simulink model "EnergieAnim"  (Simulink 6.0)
settings: Solver=ode45  StartTime=0.0  StopTime=SimTime  FixedStep=1E-2  RelTol=1e-5
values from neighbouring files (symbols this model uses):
  b = S/Sm    (= 0.1)    [Constantes.m]    (also in ConstantesBck.m)
  beta = 1    [ResCourV1.m]    (also in ResCrV1.m; ResEnerV1.m; Constantes.m = 0.95; ConstantesBck.m = 0.95)
  C = 1    [Constantes.m]    (also in ConstantesBck.m)
  Cdl = 731.3E-9    (= 7.313e-07)    [ResCourV1.m]    (also in ResCrV1.m; ResEnerV1.m; Constantes.m = 6.03e-07; ConstantesBck.m = 6.03e-07)
  Cmem = 1E-6*Sm*(1-b)    (= 2.826e-08)    [Constantes.m]    (also in ConstantesBck.m = 3.14e-11; ImpedanceZtissus.m = 4e-08; Ztissus.m = 4e-08; CalculCharge.m = 1)
  Fact = 10^2    (= 100)    [Constantes.m]    (also in ConstantesBck.m)
  gk = 36    [Constantes.m]    (also in ConstantesBck.m; sim_hh.m)
  gl = 0.3    [Constantes.m]    (also in ConstantesBck.m; sim_hh.m)
  gna = 120    [Constantes.m]    (also in ConstantesBck.m; sim_hh.m)
  h0 = cdep(4)    [temps.m]    (also in Constantes.m = 0.5961; ConstantesBck.m = 0.5961)
  I0Stim = AddI    (= 0)    [WaveComp.m]    (also in WaveCompIET.m; WaveCompIETAnim.m; WaveCompIETIf.m; WaveCompIETSeul.m = Hm(i)*1E-6)
  m0 = cdep(5)    [temps.m]    (also in Constantes.m = 0.0529; ConstantesBck.m = 0.0529)
  mK = 0    [Constantes.m]    (also in ConstantesBck.m)
  mL = 0    [Constantes.m]    (also in ConstantesBck.m)
  mNa = 0    [Constantes.m]    (also in ConstantesBck.m)
  n0 = 0.3177    [Constantes.m]    (also in ConstantesBck.m)
  Rcan = 6.398E3*Sm*(1-b)    (= 180.80748)    [Constantes.m]    (also in ConstantesBck.m = 0.03454; ImpedanceZtissus.m = 44; Ztissus.m = 44)
  Rct = 605.2E3    (= 605200)    [ResCourV1.m]    (also in ResCrV1.m; ResEnerV1.m; Constantes.m = 185600; ConstantesBck.m = 185600)
  sigma = 68000    [ResCourV1.m]    (also in ResCrV1.m; ResEnerV1.m; Constantes.m = 66466; ConstantesBck.m = 66466)
  Sm = 3.14e-2    (= 0.0314)    [Constantes.m]    (also in ConstantesBck.m = 0.000314)
  T0Stim = i    [WaveComp.m]    (also in WaveCompIET.m; WaveCompIETAnim.m = 5; WaveCompIETIf.m; WaveCompIETSeul.m = T0Hm(i)*1E-3)
  TypeStim = 5    [WaveComp.m]    (also in WaveCompIET.m; WaveCompIETAnim.m; WaveCompIETIf.m; WaveCompIETSeul.m)
  Vk = -82    [Constantes.m]    (also in ConstantesBck.m)
  Vl = -59    [Constantes.m]    (also in ConstantesBck.m)
  Vna = 45    [Constantes.m]    (also in ConstantesBck.m)
  Vr = -70    [Constantes.m]    (also in ConstantesBck.m)
libraries: simulink x1

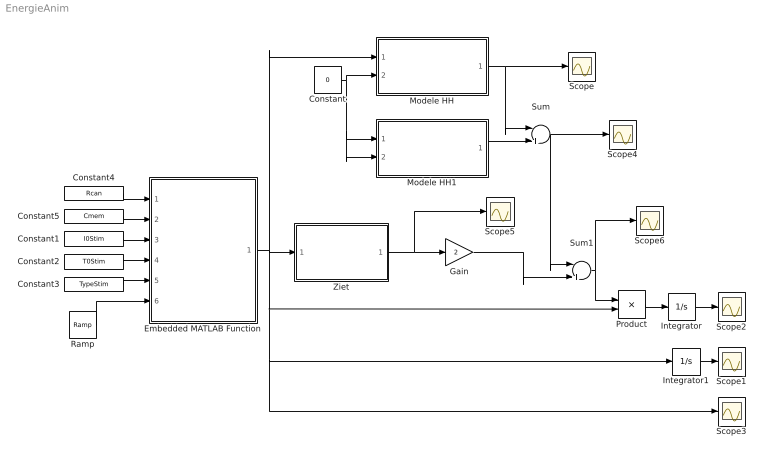
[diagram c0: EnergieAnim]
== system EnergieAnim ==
  Constant : Constant  Value=0
  Constant1 : Constant  Value=I0Stim
  Constant2 : Constant  Value=T0Stim
  Constant3 : Constant  Value=TypeStim
  Constant4 : Constant  Value=Rcan
  Constant5 : Constant  Value=Cmem
  Embedded MATLAB Function : Stateflow chart
  Gain : Gain  Gain=2
  Integrator : Integrator
  Integrator1 : Integrator
  Modele HH : Subsystem
  Modele HH1 : Subsystem
  Product : Product
  Ramp : simulink/Sources/Ramp  slope=1  start=0  X0=0
  Scope{,1..6} (7 alike) : Scope
  Sum : Sum  Inputs=|+-
  Sum1 : Sum  Inputs=|++
  Ziet : Subsystem
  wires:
  Product/1 -> Integrator/1
  Constant1/1 -> Embedded MATLAB Function/3(I0Stim)
  Constant2/1 -> Embedded MATLAB Function/4(T0Stim)
  Constant3/1 -> Embedded MATLAB Function/5(TypeStim)
  Ramp/1 -> Embedded MATLAB Function/6(temps)
  Embedded MATLAB Function/1(Istim) -> Product/2, Scope3/1, Integrator1/1, Modele HH/1(HHin), Ziet/1(InZiet)
  Constant4/1 -> Embedded MATLAB Function/1(Rcan)
  Constant5/1 -> Embedded MATLAB Function/2(Cmem)
  Modele HH/1(HHout) -> Scope/1, Sum/1
  Constant/1 -> Modele HH/2(VRefIn), Modele HH1/1(HHin), Modele HH1/2(VRefIn)
  Integrator/1 -> Scope2/1
  Modele HH1/1(HHout) -> Sum/2
  Sum/1 -> Sum1/1, Scope4/1
  Sum1/1 -> Product/1, Scope6/1
  Ziet/1(OutZiet) -> Gain/1, Scope5/1
  Gain/1 -> Sum1/2
  Integrator1/1 -> Scope1/1

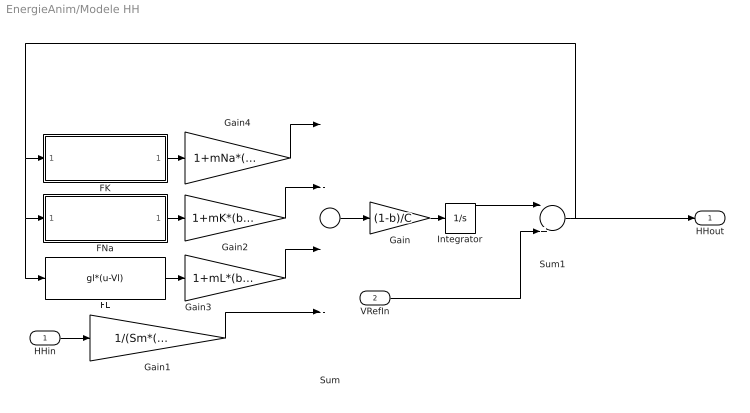
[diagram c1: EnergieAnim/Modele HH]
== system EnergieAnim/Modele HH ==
  HHin : Inport  Port=1  LatchInput=off
  VRefIn : Inport  Port=2  LatchInput=off
  FK : Subsystem
  FL : Fcn  Expr=gl*(u-Vl)
  FNa : Subsystem
  Gain : Gain  Gain=(1-b)/C
  Gain1 : Gain  Gain=1/(Sm*(1-b)*Fact)
  Gain2 : Gain  Gain=1+mK*(b/(1-b))
  Gain3 : Gain  Gain=1+mL*(b/(1-b))
  Gain4 : Gain  Gain=1+mNa*(b/(1-b))
  Integrator : Integrator  InitialCondition=Vr
  Sum : Sum  Inputs=|---+
  Sum1 : Sum  Inputs=|++
  HHout : Outport
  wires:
  Sum/1 -> Gain/1
  Gain/1 -> Integrator/1
  FK/1(FKout) -> Gain4/1
  FNa/1(FNaOut) -> Gain2/1
  FL/1 -> Gain3/1
  HHin/1 -> Gain1/1
  Integrator/1 -> Sum1/1
  Sum1/1 -> FNa/1(FNaIn), FL/1, FK/1(FKIn), HHout/1
  Gain1/1 -> Sum/4
  Gain4/1 -> Sum/1
  Gain2/1 -> Sum/2
  Gain3/1 -> Sum/3
  VRefIn/1 -> Sum1/2

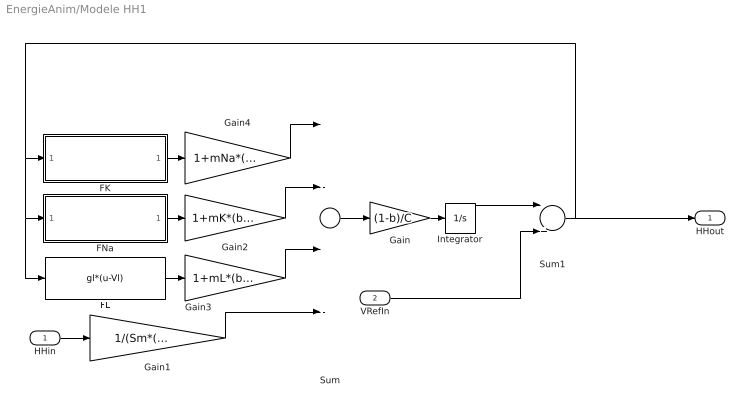
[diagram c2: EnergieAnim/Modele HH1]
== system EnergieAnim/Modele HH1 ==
  HHin : Inport  Port=1  LatchInput=off
  VRefIn : Inport  Port=2  LatchInput=off
  FK : Subsystem
  FL : Fcn  Expr=gl*(u-Vl)
  FNa : Subsystem
  Gain : Gain  Gain=(1-b)/C
  Gain1 : Gain  Gain=1/(Sm*(1-b)*Fact)
  Gain2 : Gain  Gain=1+mK*(b/(1-b))
  Gain3 : Gain  Gain=1+mL*(b/(1-b))
  Gain4 : Gain  Gain=1+mNa*(b/(1-b))
  Integrator : Integrator  InitialCondition=Vr
  Sum : Sum  Inputs=|---+
  Sum1 : Sum  Inputs=|++
  HHout : Outport
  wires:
  Sum/1 -> Gain/1
  Gain/1 -> Integrator/1
  FK/1(FKout) -> Gain4/1
  FNa/1(FNaOut) -> Gain2/1
  FL/1 -> Gain3/1
  HHin/1 -> Gain1/1
  Integrator/1 -> Sum1/1
  Sum1/1 -> FNa/1(FNaIn), FL/1, FK/1(FKIn), HHout/1
  Gain1/1 -> Sum/4
  Gain4/1 -> Sum/1
  Gain2/1 -> Sum/2
  Gain3/1 -> Sum/3
  VRefIn/1 -> Sum1/2

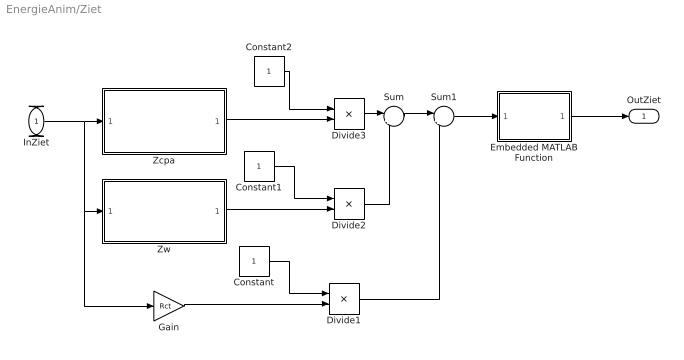
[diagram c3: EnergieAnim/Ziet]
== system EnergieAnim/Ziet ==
  InZiet : Inport  Port=1  LatchInput=off
  Constant : Constant
  Constant1 : Constant
  Constant2 : Constant
  Divide1 : Product  Inputs=*/  OutScaling=2^-10
  Divide2 : Product  Inputs=*/  OutScaling=2^-10
  Divide3 : Product  Inputs=*/  OutScaling=2^-10
  Embedded MATLAB Function : Stateflow chart
  Gain : Gain  Gain=Rct
  Sum : Sum  Inputs=|++
  Sum1 : Sum  Inputs=|++
  Zcpa : Subsystem
  Zw : Subsystem
  OutZiet : Outport
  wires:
  Constant/1 -> Divide1/1
  Constant1/1 -> Divide2/1
  Constant2/1 -> Divide3/1
  Zcpa/1(OutZcpa) -> Divide3/2
  Zw/1(OutZw) -> Divide2/2
  Divide3/1 -> Sum/1
  Divide2/1 -> Sum/2
  Sum/1 -> Sum1/1
  Divide1/1 -> Sum1/2
  Sum1/1 -> Embedded MATLAB Function/1(u)
  Gain/1 -> Divide1/2
  InZiet/1 -> Zcpa/1(InZcpa), Zw/1(InZw), Gain/1
  Embedded MATLAB Function/1(y) -> OutZiet/1

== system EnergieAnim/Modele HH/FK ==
  note: gkm
  note: (Vm-Vk0)
  FKIn : Inport  Port=1  LatchInput=off
  (Vm-Vk0) : Fcn  Expr=(u-Vk)
  Product : Product
  n(Vm) : Subsystem
  n^4 : Fcn  Expr=gk*(u^4)
  FKout : Outport  InitialOutput=0
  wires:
  n(Vm)/1(n) -> n^4/1
  (Vm-Vk0)/1 -> Product/2
  Product/1 -> FKout/1
  n^4/1 -> Product/1
  FKIn/1 -> n(Vm)/1(Vm), (Vm-Vk0)/1

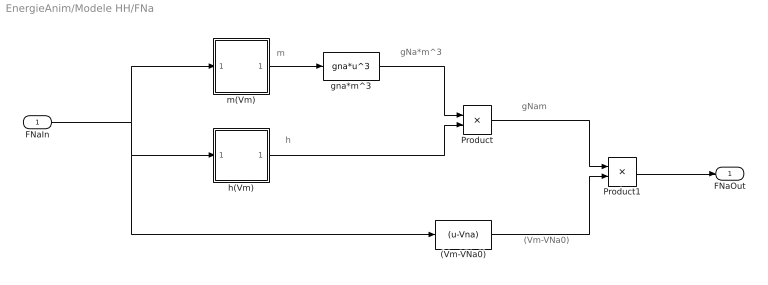
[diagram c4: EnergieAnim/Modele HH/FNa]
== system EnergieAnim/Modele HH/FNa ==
  note: gNa*m^3
  note: m
  note: h
  note: gNam
  note: (Vm-VNa0)
  FNaIn : Inport  Port=1  LatchInput=off
  (Vm-VNa0) : Fcn  Expr=(u-Vna)
  Product : Product
  Product1 : Product
  gna*m^3 : Fcn  Expr=gna*u^3
  h(Vm) : Subsystem
  m(Vm) : Subsystem
  FNaOut : Outport  InitialOutput=0
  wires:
  (Vm-VNa0)/1 -> Product1/2
  gna*m^3/1 -> Product/1
  Product1/1 -> FNaOut/1
  FNaIn/1 -> m(Vm)/1(Vm), h(Vm)/1(Vm), (Vm-VNa0)/1
  m(Vm)/1(n) -> gna*m^3/1
  h(Vm)/1(h) -> Product/2
  Product/1 -> Product1/1

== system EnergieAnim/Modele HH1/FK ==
  note: gkm
  note: (Vm-Vk0)
  FKIn : Inport  Port=1  LatchInput=off
  (Vm-Vk0) : Fcn  Expr=(u-Vk)
  Product : Product
  n(Vm) : Subsystem
  n^4 : Fcn  Expr=gk*(u^4)
  FKout : Outport  InitialOutput=0
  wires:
  n(Vm)/1(n) -> n^4/1
  (Vm-Vk0)/1 -> Product/2
  Product/1 -> FKout/1
  n^4/1 -> Product/1
  FKIn/1 -> n(Vm)/1(Vm), (Vm-Vk0)/1

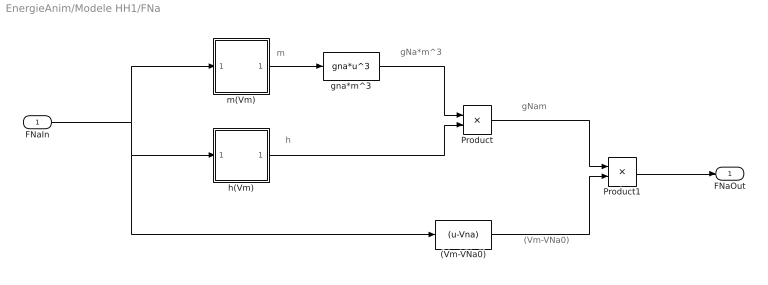
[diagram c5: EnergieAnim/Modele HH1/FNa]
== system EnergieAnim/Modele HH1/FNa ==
  note: gNa*m^3
  note: m
  note: h
  note: gNam
  note: (Vm-VNa0)
  FNaIn : Inport  Port=1  LatchInput=off
  (Vm-VNa0) : Fcn  Expr=(u-Vna)
  Product : Product
  Product1 : Product
  gna*m^3 : Fcn  Expr=gna*u^3
  h(Vm) : Subsystem
  m(Vm) : Subsystem
  FNaOut : Outport  InitialOutput=0
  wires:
  (Vm-VNa0)/1 -> Product1/2
  gna*m^3/1 -> Product/1
  Product1/1 -> FNaOut/1
  FNaIn/1 -> m(Vm)/1(Vm), h(Vm)/1(Vm), (Vm-VNa0)/1
  m(Vm)/1(n) -> gna*m^3/1
  h(Vm)/1(h) -> Product/2
  Product/1 -> Product1/1

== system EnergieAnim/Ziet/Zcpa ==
  InZcpa : Inport  Port=1  LatchInput=off
  Fcn : Fcn  Expr=u(1)^beta
  Transfer Fcn : TransferFcn  Denominator=[Cdl 0]
  OutZcpa : Outport
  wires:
  Transfer Fcn/1 -> Fcn/1
  InZcpa/1 -> Transfer Fcn/1
  Fcn/1 -> OutZcpa/1

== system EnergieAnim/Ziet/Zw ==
  InZw : Inport  Port=1  LatchInput=off
  Gain : Gain  Gain=sigma
  Math Function : Math  Operator=sqrt
  Transfer Fcn : TransferFcn  Numerator=[2]  Denominator=[1 0]
  OutZw : Outport
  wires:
  Transfer Fcn/1 -> Math Function/1
  Math Function/1 -> Gain/1
  Gain/1 -> OutZw/1
  InZw/1 -> Transfer Fcn/1

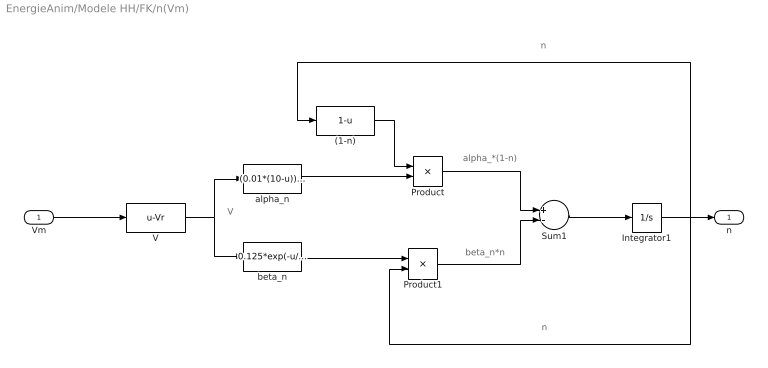
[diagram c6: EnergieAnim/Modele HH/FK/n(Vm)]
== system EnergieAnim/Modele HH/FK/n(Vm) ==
  note: V
  note: alpha_*(1-n)
  note: beta_n*n
  note: n
  note: n
  Vm : Inport  Port=1  LatchInput=off
  (1-n) : Fcn  Expr=1-u
  Integrator1 : Integrator  InitialCondition=n0
  Product : Product
  Product1 : Product
  Sum1 : Sum  Inputs=+-
  V : Fcn  Expr=u-Vr
  alpha_n : Fcn  Expr=(0.01*(10-u))/(exp((10-u)/10)-1)
  beta_n : Fcn  Expr=0.125*exp(-u/80)
  n : Outport  InitialOutput=0
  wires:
  V/1 -> alpha_n/1, beta_n/1
  alpha_n/1 -> Product/2
  (1-n)/1 -> Product/1
  beta_n/1 -> Product1/1
  Product/1 -> Sum1/1
  Product1/1 -> Sum1/2
  Sum1/1 -> Integrator1/1
  Integrator1/1 -> (1-n)/1, Product1/2, n/1
  Vm/1 -> V/1

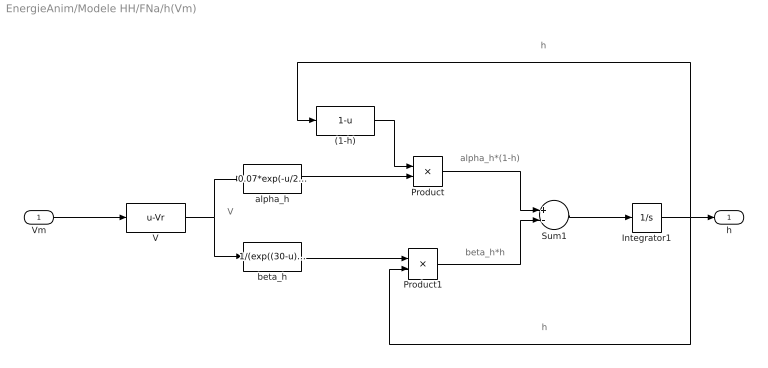
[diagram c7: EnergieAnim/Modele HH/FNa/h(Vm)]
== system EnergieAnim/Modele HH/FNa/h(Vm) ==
  note: h
  note: h
  note: beta_h*h
  note: alpha_h*(1-h)
  note: V
  Vm : Inport  Port=1  LatchInput=off
  (1-h) : Fcn  Expr=1-u
  Integrator1 : Integrator  InitialCondition=h0
  Product : Product
  Product1 : Product
  Sum1 : Sum  Inputs=+-
  V : Fcn  Expr=u-Vr
  alpha_h : Fcn  Expr=0.07*exp(-u/20)
  beta_h : Fcn  Expr=1/(exp((30-u)/10)+1)
  h : Outport  InitialOutput=0
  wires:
  Vm/1 -> V/1
  Integrator1/1 -> h/1, Product1/2, (1-h)/1
  Sum1/1 -> Integrator1/1
  Product1/1 -> Sum1/2
  Product/1 -> Sum1/1
  beta_h/1 -> Product1/1
  (1-h)/1 -> Product/1
  alpha_h/1 -> Product/2
  V/1 -> beta_h/1, alpha_h/1

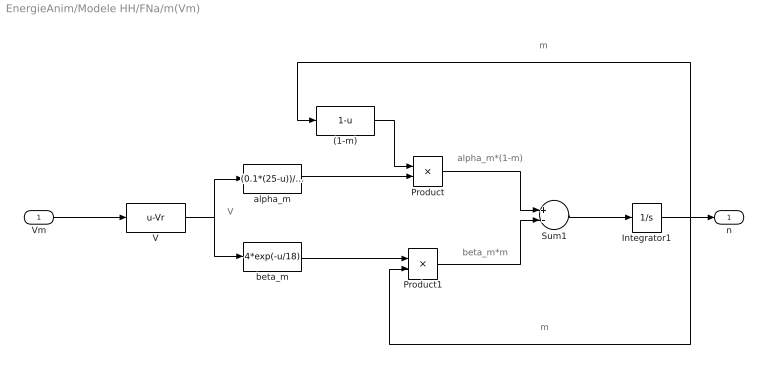
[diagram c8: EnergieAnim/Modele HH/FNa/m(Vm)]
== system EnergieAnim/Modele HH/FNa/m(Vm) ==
  note: m
  note: m
  note: beta_m*m
  note: alpha_m*(1-m)
  note: V
  Vm : Inport  Port=1  LatchInput=off
  (1-m) : Fcn  Expr=1-u
  Integrator1 : Integrator  InitialCondition=m0
  Product : Product
  Product1 : Product
  Sum1 : Sum  Inputs=+-
  V : Fcn  Expr=u-Vr
  alpha_m : Fcn  Expr=(0.1*(25-u))/(exp((25-u)/10)-1)
  beta_m : Fcn  Expr=4*exp(-u/18)
  n : Outport  InitialOutput=0
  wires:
  Vm/1 -> V/1
  Integrator1/1 -> n/1, Product1/2, (1-m)/1
  Sum1/1 -> Integrator1/1
  Product1/1 -> Sum1/2
  Product/1 -> Sum1/1
  beta_m/1 -> Product1/1
  (1-m)/1 -> Product/1
  alpha_m/1 -> Product/2
  V/1 -> beta_m/1, alpha_m/1

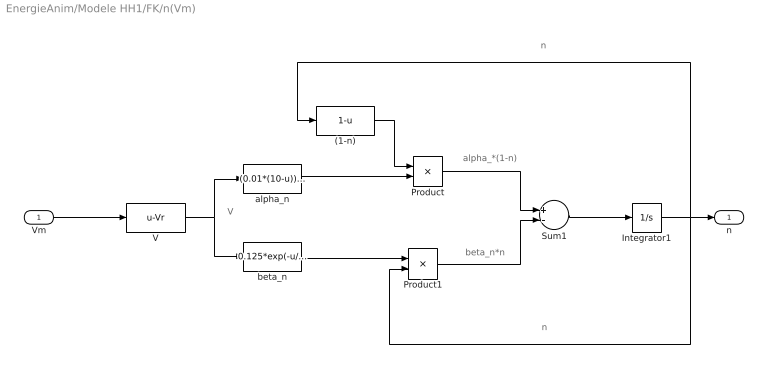
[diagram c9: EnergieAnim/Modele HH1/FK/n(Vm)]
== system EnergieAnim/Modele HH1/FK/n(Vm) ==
  note: V
  note: alpha_*(1-n)
  note: beta_n*n
  note: n
  note: n
  Vm : Inport  Port=1  LatchInput=off
  (1-n) : Fcn  Expr=1-u
  Integrator1 : Integrator  InitialCondition=n0
  Product : Product
  Product1 : Product
  Sum1 : Sum  Inputs=+-
  V : Fcn  Expr=u-Vr
  alpha_n : Fcn  Expr=(0.01*(10-u))/(exp((10-u)/10)-1)
  beta_n : Fcn  Expr=0.125*exp(-u/80)
  n : Outport  InitialOutput=0
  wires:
  V/1 -> alpha_n/1, beta_n/1
  alpha_n/1 -> Product/2
  (1-n)/1 -> Product/1
  beta_n/1 -> Product1/1
  Product/1 -> Sum1/1
  Product1/1 -> Sum1/2
  Sum1/1 -> Integrator1/1
  Integrator1/1 -> (1-n)/1, Product1/2, n/1
  Vm/1 -> V/1

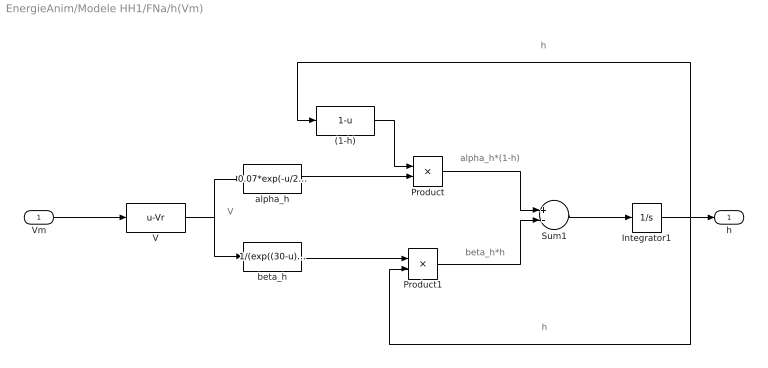
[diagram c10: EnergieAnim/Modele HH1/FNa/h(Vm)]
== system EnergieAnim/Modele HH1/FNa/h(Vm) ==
  note: h
  note: h
  note: beta_h*h
  note: alpha_h*(1-h)
  note: V
  Vm : Inport  Port=1  LatchInput=off
  (1-h) : Fcn  Expr=1-u
  Integrator1 : Integrator  InitialCondition=h0
  Product : Product
  Product1 : Product
  Sum1 : Sum  Inputs=+-
  V : Fcn  Expr=u-Vr
  alpha_h : Fcn  Expr=0.07*exp(-u/20)
  beta_h : Fcn  Expr=1/(exp((30-u)/10)+1)
  h : Outport  InitialOutput=0
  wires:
  Vm/1 -> V/1
  Integrator1/1 -> h/1, Product1/2, (1-h)/1
  Sum1/1 -> Integrator1/1
  Product1/1 -> Sum1/2
  Product/1 -> Sum1/1
  beta_h/1 -> Product1/1
  (1-h)/1 -> Product/1
  alpha_h/1 -> Product/2
  V/1 -> beta_h/1, alpha_h/1

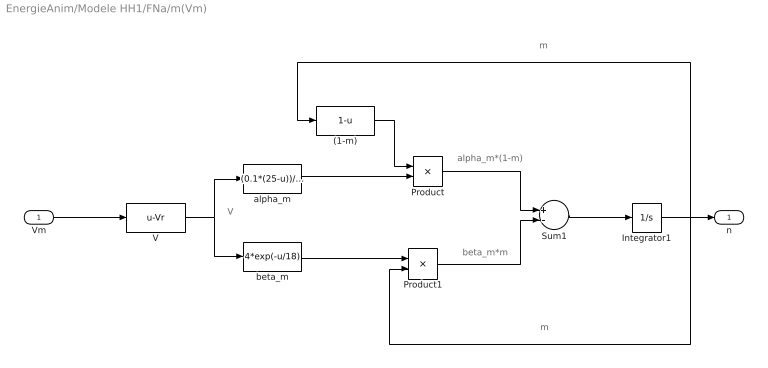
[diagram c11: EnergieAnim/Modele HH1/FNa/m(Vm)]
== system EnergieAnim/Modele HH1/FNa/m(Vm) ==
  note: m
  note: m
  note: beta_m*m
  note: alpha_m*(1-m)
  note: V
  Vm : Inport  Port=1  LatchInput=off
  (1-m) : Fcn  Expr=1-u
  Integrator1 : Integrator  InitialCondition=m0
  Product : Product
  Product1 : Product
  Sum1 : Sum  Inputs=+-
  V : Fcn  Expr=u-Vr
  alpha_m : Fcn  Expr=(0.1*(25-u))/(exp((25-u)/10)-1)
  beta_m : Fcn  Expr=4*exp(-u/18)
  n : Outport  InitialOutput=0
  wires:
  Vm/1 -> V/1
  Integrator1/1 -> n/1, Product1/2, (1-m)/1
  Sum1/1 -> Integrator1/1
  Product1/1 -> Sum1/2
  Product/1 -> Sum1/1
  beta_m/1 -> Product1/1
  (1-m)/1 -> Product/1
  alpha_m/1 -> Product/2
  V/1 -> beta_m/1, alpha_m/1

== matlab function Ziet/Embedded
MATLAB Function ==
function y = fcn(u)
% This block supports an embeddable subset of the MATLAB language.
% See the help menu for details. 

if u == Inf 
    y = 0;
else
    y = 1/u;
end

== matlab function Embedded
MATLAB Function ==
function Istim = courant(Rcan,Cmem,I0Stim,T0Stim,TypeStim,temps)
% This block supports an embeddable subset of the MATLAB language.
% See the help menu for details. 
taum = 1/30.4E-3*1E-6*1000;
if temps <= T0Stim
    if TypeStim == 0
        Iout = I0Stim;
    elseif TypeStim == 1
        Iout = I0Stim*exp(temps/taum);
    elseif TypeStim == 2
        Iout = I0Stim*sin(pi/T0Stim*temps);
    elseif TypeStim == 3
        Iout = I0Stim*sin(pi/(2*T0Stim)*temps);
    elseif TypeStim == 4
        Iout = I0Stim*sinh(temps/taum);
    else
        Iout = I0Stim*(sin(pi/T0Stim*temps)+1/3*sin(3*pi/T0Stim*temps));
    end
else
    Iout = 0;
end
Istim = Iout;
